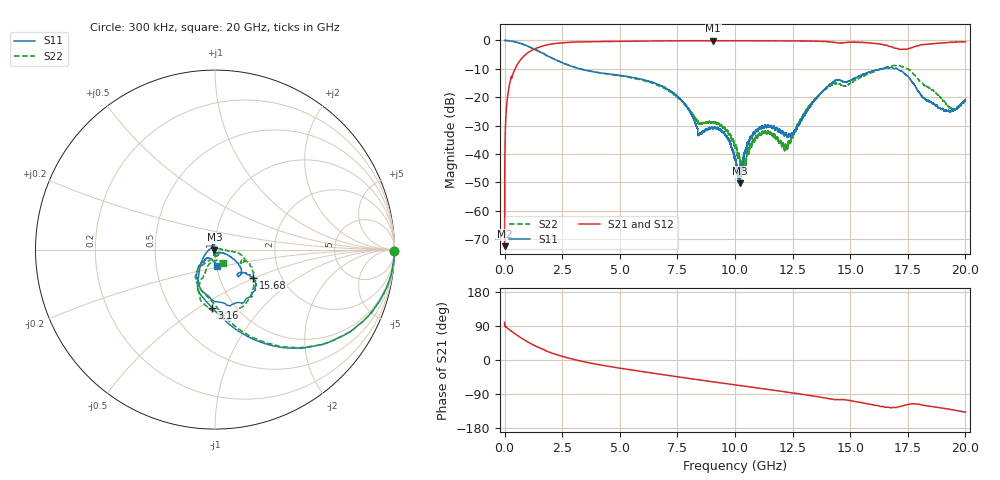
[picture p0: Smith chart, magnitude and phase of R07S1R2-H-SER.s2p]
!{R07S1R2}
!Johanson Technology Inc.
!www.johansontechnology.com
!Test Board Conditions:
!Substrate Type  RO4350B
!Substrate Thickness  10 mil
!Substrate Dk  3.66
!TL Type: GCPW
!TL Trace Width  21 mil
!TL Gap  20 mil
!Electrode orientation  Horizontal
!DUT TOPOLOGY	SERIES
!Mounting Pad LxW  16x21 mil
! Created Fri Feb  5 23:10:49 2021
# hz S ma R 50
! 2 Port Network Data from SP1.SP block
! freq  magS11  angS11  magS21  angS21  magS12  angS12  magS22  angS22
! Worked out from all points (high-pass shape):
!   20001 points, 300 kHz to 20 GHz, reference 50 ohm
!   highest |S21| = -0.08 dB at 9.058 GHz (marker M1); lowest = -72.5 dB at 300 kHz (marker M2)
!   |S21| within 3 dB of the highest: 1.279 GHz to 17.13 GHz (15.85 GHz wide, 172 % of centre); 17.46 GHz to end of sweep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
!   lowest |S11| = -50.4 dB at 10.21 GHz (marker M3), VSWR 1.01, Z = 49.7 - j0.0331 ohm
!   |S11| at or under -10 dB: 3.247713 GHz to 3.249209 GHz (1.496 MHz wide, 0.0461 % of centre); 3.249 GHz to 16.3 GHz (13.05 GHz wide, 134 % of centre); 17.05 GHz to end of sweep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
!   |S22| runs from -46.0 to 0.0 dB; largest |S21 - S12| = 0.014
!   S11 on the Smith chart (normalised r, x): 300 kHz: open; 3.16 GHz: 0.79, -0.57; 15.68 GHz: 1.44, -0.48; 20 GHz: 1.01, -0.18
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300000  0.9998 -0.5  0.0002359 99.2  0.0002543 95.5  1 -0.6
1.323e8  0.994 -6.8  0.1061 83.4  0.106 83.6  0.9936 -6.8
4.933e8  0.9366 -22.2  0.3391 67.5  0.339 67.3  0.9384 -22.0
1.8503e9  0.5363 -67.5  0.8378 22.7  0.8376 22.8  0.5383 -66.2
3.1603e9  0.3233 -92.9  0.9417 -0.7  0.9404 -0.8  0.328 -87.5
3.3343e9  0.3098 -95.7  0.9456 -3.2  0.9454 -3.2  0.3134 -89.5
6.6673e9  0.1682 -122.8  0.9796 -36.8  0.9797 -36.8  0.1611 -129.4
7.7593e9  0.08094 -144.6  0.9871 -46.5  0.9868 -46.6  0.0798 -122.6
8.4793e9  0.02308 145.9  0.9888 -52.7  0.9898 -52.8  0.03464 -79.6
9.0583e9  0.02753 111.2  0.9911 -57.7  0.9901 -57.8  0.03541 -57.8
9.5903e9  0.0207 103.9  0.9891 -62.1  0.9886 -62.2  0.02623 -57.0
1.00003e10  0.008419 121.9  0.9897 -65.6  0.9894 -65.7  0.01271 -74.7
1.02133e10  0.00301 -173.6  0.9874 -67.4  0.9869 -67.4  0.007626 -97.0
1.08653e10  0.02245 -106.4  0.9881 -72.7  0.9863 -72.8  0.01799 141.4
1.22103e10  0.02265 -77.5  0.9823 -84.4  0.9825 -84.4  0.01441 61.7
1.33343e10  0.07563 -22.7  0.9747 -94.5  0.9747 -94.6  0.07981 -5.2
1.43173e10  0.1941 -40.6  0.925 -104.5  0.9267 -104.4  0.1749 -19.1
1.56833e10  0.2631 -36.5  0.9145 -114.8  0.9157 -114.8  0.2494 -30.7
1.66673e10  0.3248 -56.2  0.7896 -124.8  0.7928 -125.4  0.3472 -60.5
1.76373e10  0.1975 -119.5  0.7359 -116.0  0.7345 -116.1  0.2885 -106.6
1.90223e10  0.06275 -128.1  0.9045 -127.1  0.9041 -127.4  0.08711 -112.2
2e10  0.0907 -82.2  0.9478 -137.7  0.9434 -137.7  0.08779 -58.0
